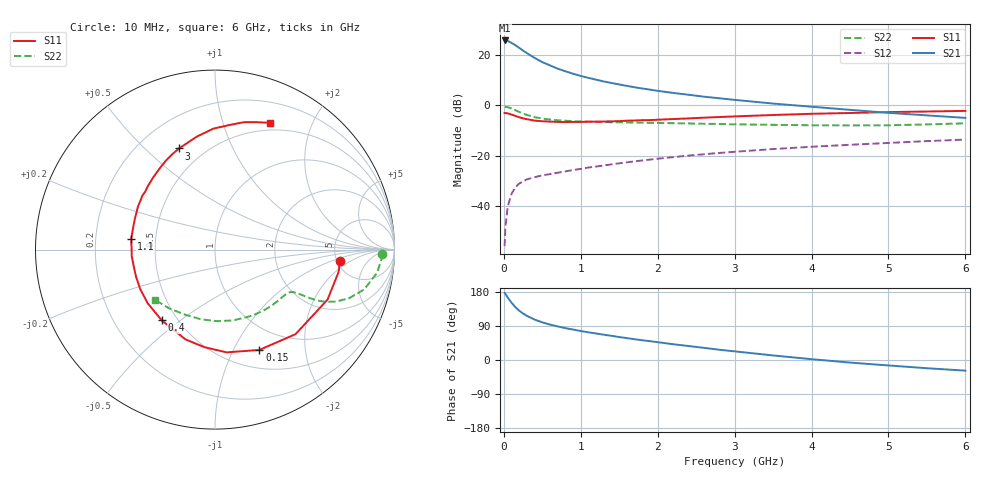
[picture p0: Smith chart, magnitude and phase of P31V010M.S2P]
! SIEMENS Small Signal Semiconductors
! BFP181
! Si NPN RF Bipolar Junction Transistor in SOT143
! VCE = 1 V  IC = 10 mA
! Common Emitter S-Parameters:  March  1996
# GHz  S  MA  R  50
!  f  S11  S21  S12  S22
! GHz  MAG  ANG  MAG  ANG  MAG  ANG  MAG  ANG
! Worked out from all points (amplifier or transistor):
!   36 points, 10 MHz to 6 GHz, reference 50 ohm
!   highest |S21| = 25.7 dB at 10 MHz (marker M1)
!   |S21| within 3 dB of that: start of sweep to 202.9 MHz
!   unconditionally stable (mu >= 1): start of sweep to 11 MHz; 573.8 MHz to end of sweep
!   at 250 MHz: K = 0.54, MSG = 25.9 dB, |S12| = -30.2 dB
!   at 1.4 GHz: K = 1.53, MAG = 11.8 dB, |S12| = -23.5 dB
!   at 6 GHz: K = 1.33, MAG = 0.9 dB, |S12| = -13.7 dB
!   S11 on the Smith chart (normalised r, x): 10 MHz: 5.30, -1.28; 150 MHz: 0.71, -1.27; 400 MHz: 0.41, -0.43; 1.1 GHz: 0.36, +0.06; 3 GHz: 0.36, +0.64; 6 GHz: 0.42, +1.44
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0.01  0.6978 -5.1  19.17 177.0  0.0016 85.1  0.9322 -1.5
0.02  0.7001 -10.1  19.15 174.3  0.0038 83.2  0.9291 -3.2
0.05  0.6862 -24.0  18.78 164.9  0.0096 78.5  0.9126 -8.1
0.1  0.6506 -46.4  17.14 151.3  0.0175 68.2  0.8599 -15.0
0.15  0.6113 -66.1  15.44 139.5  0.0236 59.8  0.7937 -20.0
0.2  0.5763 -83.5  13.67 130.1  0.0279 54.6  0.7332 -23.3
0.25  0.5468 -96.2  12.06 122.6  0.0308 50.2  0.68 -25.3
0.3  0.5267 -108.2  10.74 116.6  0.0338 47.7  0.6395 -26.4
0.4  0.4933 -127.0  8.651 106.6  0.0373 45.2  0.5787 -27.3
0.5  0.4796 -141.3  7.136 99.3  0.0405 43.3  0.5416 -27.6
0.6  0.4713 -151.9  6.134 93.5  0.043 43.5  0.5183 -28.0
0.7  0.4653 -161.0  5.287 88.6  0.0458 43.9  0.5018 -28.4
0.9  0.4653 -175.5  4.201 80.3  0.0519 44.7  0.4814 -29.5
1.1  0.471 172.7  3.475 73.0  0.058 46.0  0.4691 -31.4
1.3  0.4733 163.5  2.944 66.7  0.0637 46.4  0.4621 -33.9
1.6  0.4918 150.7  2.411 57.8  0.0734 46.6  0.4541 -37.9
2.2  0.5297 130.5  1.748 41.7  0.0932 45.2  0.4386 -48.1
3  0.5983 109.6  1.273 22.8  0.1189 40.7  0.4165 -64.0
3.5  0.6376 99.1  1.075 12.0  0.1348 37.5  0.4073 -75.7
4.5  0.6992 83.3  0.807 -6.8  0.1638 29.6  0.3962 -101.7
5.5  0.7478 71.7  0.627 -21.7  0.1938 22.2  0.4151 -127.8
6  0.77 66.5  0.559 -28.1  0.2077 17.7  0.4366 -140.2
